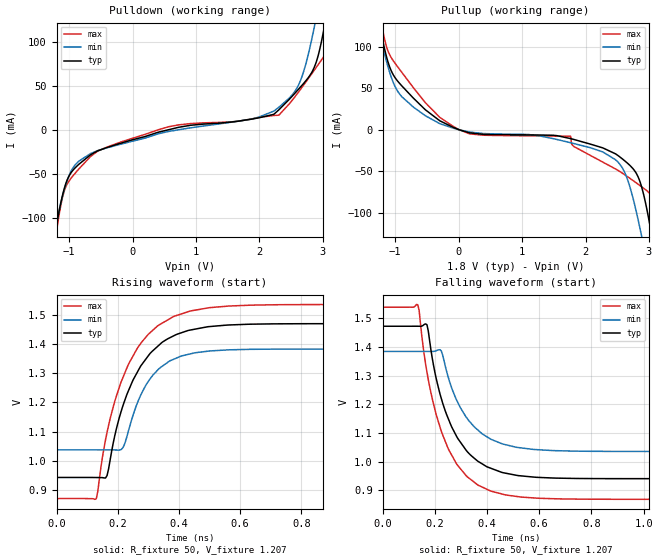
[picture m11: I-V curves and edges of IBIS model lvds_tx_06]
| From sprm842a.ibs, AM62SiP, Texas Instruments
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|   MODEL lvds_tx_06
[Model] lvds_tx_06
Model_type Output
C_comp 1.599p 1.604p 1.531p
Vmeas = 1.2
Vref = 1.2V
Rref = 50
Cref = 0.5pF
[Model Spec]
[Temperature Range]  40 150 -40
[Voltage Range] 1.8 1.62 1.98
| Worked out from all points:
|   slope of the pulldown table from 0 to 0.27 V, typ, clamps not added: 50.1 ohm
|   slope of the pullup table from 0 to 0.27 V, typ, clamps not added: 56.5 ohm
|   rising waveform, R_fixture 50, V_fixture 1.207: 20-80 % time 120ps typ, 97ps min, 127ps max; typ from 0.942 V to 1.47 V
|   falling waveform, R_fixture 50, V_fixture 1.207: 20-80 % time 125ps typ, 125ps min, 122ps max; typ from 1.47 V to 0.941 V
[Pulldown]
-1.715V   -358.7mA   -310.8mA   -423mA
-1.208V   -111.5mA   -107.5mA   -119.4mA
-1.102V   -73.47mA   -74.47mA   -75.91mA
-1.007V   -53.14mA   -52.82mA   -58.67mA
-552.1mV  -23.99mA   -23.72mA   -24.36mA
566.3mV   0A         -1.945mA   3.398mA
2.308V    22.83mA    25.67mA    16.76mA
2.631V    47.3mA     53.2mA     44.33mA
2.864V    70.85mA    116.3mA    67.64mA
3.017V    114.7mA    174.2mA    83.51mA
3.175V    184.1mA    238.9mA    118.9mA
3.514V    352.3mA    380.7mA    306.4mA
[Pullup]
-1.714V   352.3mA    305.2mA    416.7mA
-1.27V    136.2mA    125.7mA    153.2mA
-989.5mV  61.13mA    49.91mA    78.44mA
-524.2mV  23.91mA    16.78mA    32.42mA
168.5mV   -3.718mA   -2.672mA   -4.862mA
1.765V    -10.66mA   -15.62mA   -7.815mA
2.474V    -28.96mA   -36.08mA   -47.15mA
2.669V    -40.72mA   -61.35mA   -56.73mA
2.886V    -69.06mA   -128.4mA   -68.6mA
3.045V    -127.2mA   -190mA     -79.54mA
3.188V    -193.6mA   -248.8mA   -122.5mA
3.515V    -358.7mA   -386.4mA   -311.5mA
[Ramp]
dV/dt_r .318/120.259p .208/96.978p .401/126.832p
dV/dt_f .318/124.546p .208/124.542p .401/122.194p
[Rising Waveform]
R_fixture = 50
V_fixture = 1.207
V_fixture_min = 1.21
V_fixture_max = 1.204
0s        941.7mV    1.037V     869mV
130ps     941.4mV    1.037V     868.2mV
165ps     948mV      1.037V     1.097V
190ps     1.084V     1.036V     1.204V
215ps     1.183V     1.042V     1.281V
235ps     1.241V     1.102V     1.332V
295ps     1.354V     1.265V     1.429V
385ps     1.431V     1.35V      1.497V
630ps     1.47V      1.383V     1.535V
1.525ns   1.472V     1.384V     1.538V
[Falling Waveform]
R_fixture = 50
V_fixture = 1.207
V_fixture_min = 1.21
V_fixture_max = 1.204
0s        1.472V     1.384V     1.538V
135ps     1.472V     1.384V     1.547V
170ps     1.477V     1.384V     1.312V
200ps     1.313V     1.385V     1.183V
225ps     1.22V      1.385V     1.106V
280ps     1.094V     1.222V     997.9mV
365ps     1.002V     1.11V      918.6mV
460ps     961.9mV    1.062V     886.8mV
580ps     946.3mV    1.042V     873.7mV
1.525ns   941.1mV    1.036V     868.9mV
